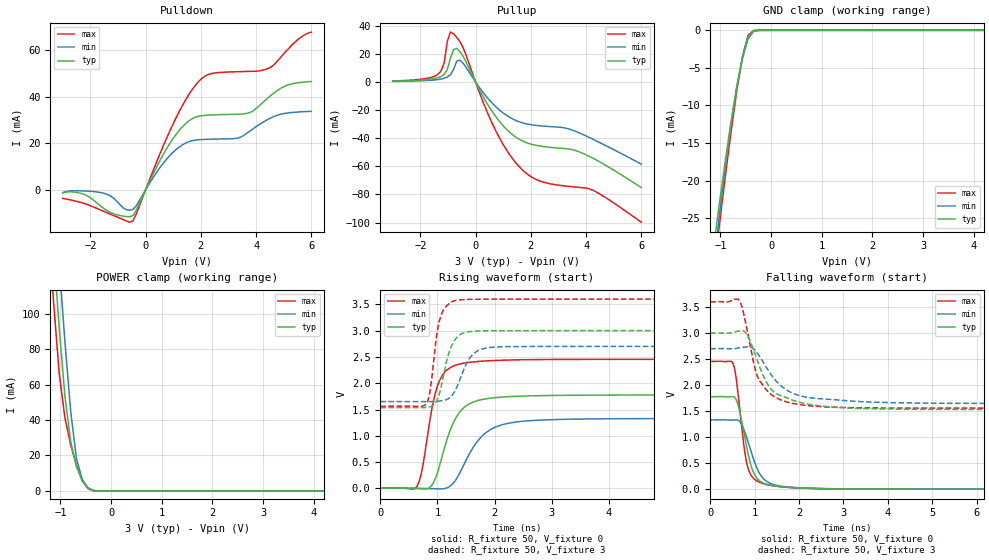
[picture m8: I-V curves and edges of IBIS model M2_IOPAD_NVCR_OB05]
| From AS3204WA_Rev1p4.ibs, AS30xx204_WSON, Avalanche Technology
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[Model] M2_IOPAD_NVCR_OB05
Model_type I/O
Enable   Active-High
Vinl  =  0.9
Vinh  =  2.1
Vmeas =  1.5
Cref  =  30e-12
| Capacitance  typ   min   max
C_comp   3.872127e-12   3.590660e-12   4.176448e-12
| Variables   typ   min   max
[GND Clamp Reference]   0   0   0
[POWER Clamp Reference]   3   2.7   3.6
[Pulldown Reference]   0   0   0
[Pullup Reference]   3   2.7   3.6
[Temperature Range]   25   105   -40
[Voltage Range]   3   2.7   3.6
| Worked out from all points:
|   slope of the pulldown table from 0 to 0.45 V, typ, clamps not added: 40.8 ohm
|   slope of the pullup table from 0 to 0.45 V, typ, clamps not added: 27.6 ohm
|   GND clamp passes 1 mA (typ) near -0.46 V on its own axis
|   POWER clamp passes 1 mA (typ) near -0.42 V on its own axis
|   falling waveform, R_fixture 50, V_fixture 0: 20-80 % time 277ps typ, 345ps min, 216ps max; typ from 1.78 V to 0 V
|   falling waveform, R_fixture 50, V_fixture 3: 20-80 % time 546ps typ, 667ps min, 412ps max; typ from 3 V to 1.53 V
|   rising waveform, R_fixture 50, V_fixture 0: 20-80 % time 352ps typ, 476ps min, 252ps max; typ from 0 V to 1.78 V
|   rising waveform, R_fixture 50, V_fixture 3: 20-80 % time 207ps typ, 264ps min, 149ps max; typ from 1.53 V to 3 V
[GND Clamp]
| Voltage   I(typ)   I(min)   I(max)
-3V       -145.9mA   -151.9mA   -144.2mA
-1.138V   -29.07mA   -31.55mA   -32.68mA
-1.024V   -23.24mA   -24.83mA   -26.15mA
-910.3mV  -17.69mA   -18.46mA   -19.83mA
-796.6mV  -12.47mA   -12.67mA   -13.82mA
-682.8mV  -7.718mA   -7.754mA   -8.316mA
-569mV    -3.663mA   -3.867mA   -3.675mA
-455.2mV  -839.2uA   -1.152mA   -666.1uA
-341.4mV  -35.63uA   -111.1uA   -11.17uA
-113.8mV  -8.642nA   -188.3nA   -1.888nA
6V        0A         0A         0A
[POWER Clamp]
| Voltage   I(typ)   I(min)   I(max)
-3V       949.8mA    984.2mA    923.5mA
-1.252V   183.6mA    221.4mA    154mA
-1.138V   136.7mA    174.2mA    107.6mA
-1.024V   92.09mA    128.1mA    66.35mA
-910.3mV  53.33mA    83.97mA    41.06mA
-796.6mV  27.72mA    44.75mA    25.94mA
-682.8mV  13.75mA    18.06mA    14.29mA
-569mV    5.664mA    6.605mA    5.738mA
-455.2mV  1.446mA    1.789mA    1.305mA
-341.4mV  77.09uA    287.6uA    62.73uA
-227.6mV  1.148uA    12.92uA    332nA
6V        0A         0A         0A
[Pulldown]
| Voltage   I(typ)   I(min)   I(max)
-3V       -1.372mA   -1.174mA   -3.673mA
-2.276V   -1.719mA   -449.6uA   -5.658mA
-1.593V   -7.28mA    -1.244mA   -8.842mA
-455.2mV  -11.08mA   -8.424mA   -13.32mA
931mV     20.94mA    15.44mA    26.71mA
1.448V    28.51mA    20.13mA    38.71mA
1.966V    31.8mA     21.61mA    47.19mA
2.483V    32.29mA    21.85mA    50.27mA
3.745V    33.17mA    25.04mA    51mA
4.49V     40.2mA     30.71mA    52.52mA
5.11V     44.97mA    33.04mA    60mA
6V        46.63mA    33.8mA     67.91mA
[Pullup]
| Voltage   I(typ)   I(min)   I(max)
-3V       614uA      457.8uA    721uA
-1.366V   3.083mA    1.775mA    5.453mA
-1.138V   5.465mA    2.688mA    13.53mA
-1.024V   8.949mA    3.598mA    28.86mA
-910.3mV  16.94mA    5.199mA    35.55mA
-796.6mV  23.1mA     8.957mA    34.34mA
-569mV    21.73mA    15.56mA    28.87mA
620.7mV   -21.52mA   -15.36mA   -30.19mA
1.655V    -41.5mA    -28.82mA   -61.73mA
2.379V    -45.66mA   -31.21mA   -70.78mA
3.745V    -49.64mA   -36.1mA    -74.93mA
6V        -75.17mA   -58.46mA   -99.72mA
[Ramp]
dV/dt_r   1.06555/0.352337n  0.797404/0.476082n  1.47276/0.251554n
dV/dt_f   0.880737/0.545815n  0.631103/0.666562n  1.22549/0.411725n
R_load = 50
[Falling Waveform]
R_fixture = 50
V_fixture = 0
V_fixture_min = 0
V_fixture_max = 0
| Time   V(typ)   V(min)   V(max)
0s        1.776V     1.329V     2.455V
505.8ps   1.78V      1.328V     2.427V
560.1ps   1.754V     1.332V     2.26V
632ps     1.602V     1.322V     1.785V
766.5ps   1.037V     1.129V     776.8mV
871.8ps   600.6mV    853.3mV    351.1mV
996.7ps   282.3mV    519.5mV    189.8mV
1.145ns   138.6mV    257.7mV    120.2mV
1.508ns   54.5mV     70.22mV    53.78mV
21.88ns   526.5nV    619.1nV    10.53uV
[Falling Waveform]
R_fixture = 50
V_fixture = 3
V_fixture_min = 2.7
V_fixture_max = 3.6
| Time   V(typ)   V(min)   V(max)
0s        3V         2.7V       3.6V
642.3ps   3.04V      2.716V     3.64V
727.5ps   3.044V     2.728V     3.464V
833ps     2.964V     2.734V     3.046V
1.007ns   2.601V     2.671V     2.32V
1.111ns   2.354V     2.552V     2.087V
1.462ns   1.848V     2.1V       1.768V
2.242ns   1.63V      1.759V     1.602V
4.872ns   1.534V     1.653V     1.558V
21.88ns   1.532V     1.648V     1.558V
[Rising Waveform]
R_fixture = 50
V_fixture = 0
V_fixture_min = 0
V_fixture_max = 0
| Time   V(typ)   V(min)   V(max)
0s        399.8nV    444.4nV    10.49uV
628.9ps   -2.765mV   3.151mV    19.82mV
737.1ps   -10.94mV   675.2uV    384.9mV
883.7ps   37.77mV    -4.17mV    1.395V
1.032ns   408.5mV    -9.327mV   2.035V
1.295ns   1.284V     122.2mV    2.333V
1.577ns   1.617V     690.5mV    2.4V
2.042ns   1.73V      1.178V     2.434V
2.938ns   1.767V     1.306V     2.452V
21.88ns   1.776V     1.329V     2.455V
[Rising Waveform]
R_fixture = 50
V_fixture = 3
V_fixture_min = 2.7
V_fixture_max = 3.6
| Time   V(typ)   V(min)   V(max)
0s        1.532V     1.648V     1.558V
801ps     1.539V     1.65V      1.6V
866.1ps   1.552V     1.65V      1.819V
986.3ps   1.66V      1.656V     2.905V
1.058ns   1.899V     1.665V     3.273V
1.221ns   2.638V     1.729V     3.528V
1.424ns   2.94V      2.155V     3.589V
1.679ns   2.991V     2.6V       3.597V
2.137ns   2.998V     2.694V     3.599V
21.88ns   3V         2.7V       3.6V
